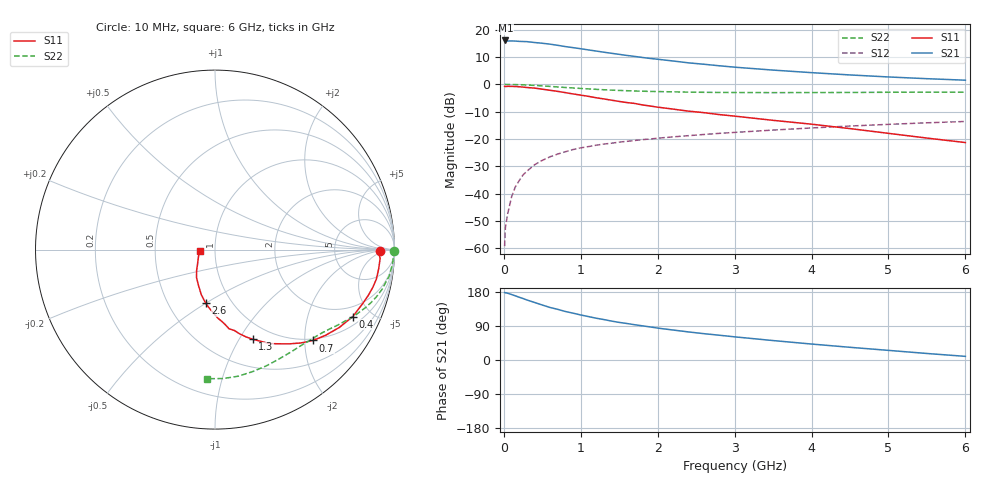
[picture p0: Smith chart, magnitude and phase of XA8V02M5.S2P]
! SIEMENS Discrete & RF Semiconductors
! BFY180
! Si NPN RF Bipolar Junction Transistor in MICRO-X
! VCE = 8 V  IC = 2.5 mA
! Common Emitter S-Parameters:  May  1997
# GHz  S  MA  R  50
!  f  S11  S21  S12  S22
! GHz  MAG  ANG  MAG  ANG  MAG  ANG  MAG  ANG
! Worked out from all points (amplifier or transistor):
!   36 points, 10 MHz to 6 GHz, reference 50 ohm
!   highest |S21| = 16.1 dB at 20 MHz (marker M1)
!   |S21| within 3 dB of that: start of sweep to 992.9 MHz
!   unconditionally stable (mu >= 1): 2.896 GHz to end of sweep
!   at 250 MHz: K = 0.13, MSG = 24.4 dB, |S12| = -33.1 dB
!   at 1.4 GHz: K = 0.69, MSG = 16.4 dB, |S12| = -21.5 dB
!   at 6 GHz: K = 1.05, MAG = 6.1 dB, |S12| = -13.6 dB
!   S11 on the Smith chart (normalised r, x): 10 MHz: 24, -2; 400 MHz: 1.41, -3.87; 700 MHz: 0.96, -2.19; 1.3 GHz: 0.81, -1.14; 2.6 GHz: 0.76, -0.50; 6 GHz: 0.84, -0.01
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0.01  0.9194 -0.5  6.319 178.0  0.0011 88.0  0.9961 -0.3
0.02  0.9133 -1.1  6.352 177.5  0.0024 92.0  0.9999 -0.7
0.05  0.9212 -3.1  6.207 176.2  0.0043 89.0  0.9949 -1.7
0.1  0.9183 -6.7  6.222 172.8  0.0087 87.2  0.9934 -3.5
0.15  0.9141 -10.3  6.19 169.3  0.0134 84.6  0.9902 -5.2
0.3  0.8764 -20.0  6.041 158.4  0.0259 77.7  0.9719 -10.2
0.4  0.8537 -25.9  5.823 151.8  0.0339 73.9  0.9575 -13.3
0.5  0.817 -32.1  5.645 145.1  0.0408 70.9  0.938 -16.2
0.6  0.7793 -37.8  5.437 138.6  0.0474 67.6  0.9178 -18.8
0.7  0.745 -42.8  5.178 133.7  0.0532 63.9  0.8972 -21.2
0.8  0.7058 -47.5  4.908 128.0  0.0586 61.8  0.8768 -23.4
1.1  0.6044 -60.0  4.264 114.6  0.0728 55.9  0.8256 -28.9
1.3  0.5418 -67.2  3.873 106.7  0.081 52.7  0.7975 -32.2
1.5  0.4872 -73.9  3.54 99.2  0.0878 50.3  0.7746 -35.0
1.7  0.4482 -79.9  3.248 93.1  0.0941 48.4  0.7564 -37.7
2  0.3829 -87.5  2.881 84.2  0.1036 45.8  0.7387 -41.6
2.2  0.3528 -91.5  2.675 79.1  0.1097 44.2  0.7297 -44.2
2.6  0.304 -99.7  2.334 69.5  0.1212 41.4  0.7159 -49.1
3.5  0.2199 -114.7  1.824 51.3  0.146 35.3  0.706 -60.0
4.5  0.1553 -131.3  1.487 33.5  0.173 28.3  0.7113 -72.7
5.5  0.1042 -153.5  1.27 17.2  0.1982 20.6  0.7199 -86.5
6  0.0863 -175.6  1.192 9.6  0.2097 16.3  0.7206 -93.4
